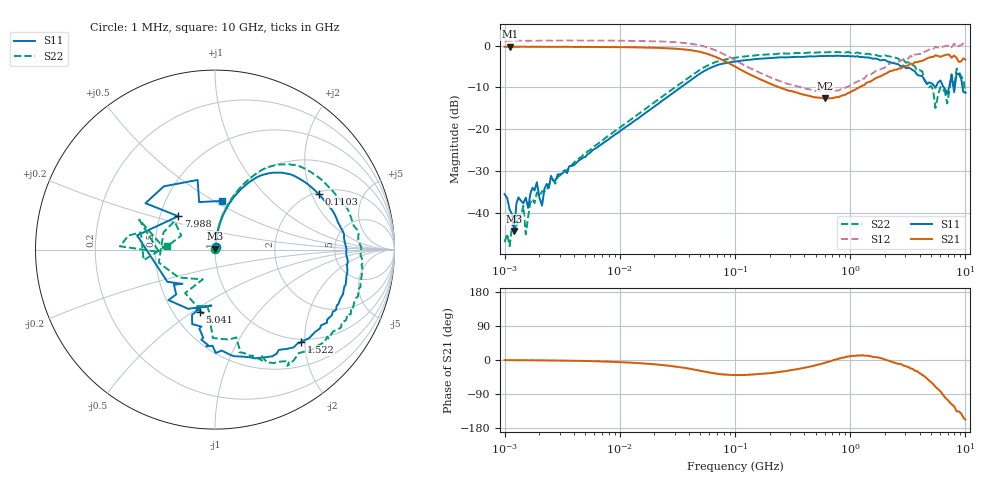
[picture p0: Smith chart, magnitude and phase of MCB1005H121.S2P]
!Agilent Technologies,E5071C,MY46111244,A.11.31
!Date: Tue May 07 16:36:44 2019
!Data & Calibration Information:
!Freq	S11:SOLT2(ON)	S21:SOLT2(ON)	S12:SOLT2(ON)	S22:SOLT2(ON)
# Hz S dB R 50
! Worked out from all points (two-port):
!   201 points, 1 MHz to 10 GHz, reference 50 ohm
!   highest |S21| = -0.29 dB at 1.106 MHz (marker M1); lowest = -12.6 dB at 610.4 MHz (marker M2)
!   |S21| within 3 dB of the highest: start of sweep to 75.69 MHz; 4.492 GHz to 8.526 GHz (4.034 GHz wide, 62 % of centre)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
!   lowest |S11| = -44.3 dB at 1.212 MHz (marker M3), VSWR 1.01, Z = 49.9 + j0.593 ohm
!   |S11| at or under -10 dB: start of sweep to 33.76 MHz; 6.505 GHz to 7.226 GHz (720 MHz wide, 10.5 % of centre); 9.458 GHz to end of sweep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
!   |S22| runs from -47.9 to -1.5 dB; largest |S21 - S12| = 0.49
!   S11 on the Smith chart (normalised r, x): 1 MHz: 1.01, +0.03; 110.3 MHz: 2.10, +2.27; 1.522 GHz: 0.94, -1.92; 5.041 GHz: 0.68, -0.53; 7.988 GHz: 0.62, +0.25; 10 GHz: 0.93, +0.54
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1000000  -35.50 65.7  -0.31 -0.3  1.13 -1.2  -46.95 58.1
1106086  -39.18 108.5  -0.29 -0.5  1.13 -1.2  -47.92 28.1
1212171  -44.27 103.5  -0.30 -0.4  1.17 -1.3  -41.92 23.4
1318257  -36.26 73.9  -0.30 -0.4  1.13 -1.4  -40.50 67.0
1453604  -37.68 72.6  -0.32 -0.5  1.15 -1.4  -38.27 84.9
1526823  -36.32 73.1  -0.29 -0.7  1.16 -1.4  -45.08 57.9
1905461  -32.65 101.2  -0.31 -0.9  1.13 -1.7  -35.12 79.8
2112549  -38.22 100.3  -0.31 -1.1  1.16 -1.9  -34.81 87.2
4810209  -26.73 85.3  -0.34 -2.5  1.18 -3.3  -26.12 83.2
2.206931e7  -13.71 76.3  -0.57 -12.6  0.99 -12.9  -12.68 75.5
1.047129e8  -3.75 29.9  -5.32 -39.9  -3.77 -39.8  -2.84 29.6
1.102671e8  -3.66 28.0  -5.67 -39.8  -4.13 -39.9  -2.75 27.4
4.810209e8  -2.62 -6.6  -12.32 -15.5  -10.75 -14.4  -1.72 -6.1
6.103625e8  -2.51 -12.3  -12.62 -7.0  -11.10 -5.2  -1.61 -11.3
1.52211e9  -3.05 -47.0  -8.52 9.3  -6.88 13.8  -2.16 -44.1
2.206931e9  -3.97 -71.6  -6.12 -2.8  -4.26 3.0  -2.61 -57.0
5.041477e9  -8.99 -103.6  -2.75 -58.7  -0.98 -47.1  -9.62 -107.9
5.495409e9  -10.11 -93.6  -2.32 -70.7  -0.26 -57.6  -14.93 -112.3
6.661376e9  -10.43 -139.5  -2.26 -99.1  -0.17 -82.8  -11.19 145.1
7.988146e9  -11.16 137.8  -2.39 -122.2  0.46 -105.5  -10.11 -177.6
8.390517e9  -6.64 146.3  -2.96 -135.6  -0.40 -115.5  -5.51 178.0
1e10  -11.25 82.0  -3.35 -157.5  0.63 -137.5  -11.44 175.3
